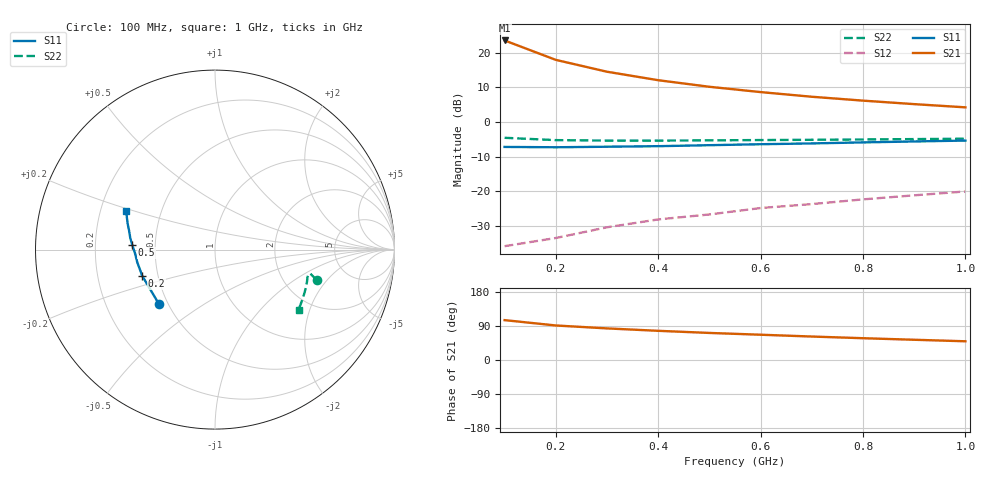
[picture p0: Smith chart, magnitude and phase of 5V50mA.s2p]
#  HZ  S  MA  R  50.0000
! Device:15GN03CA
! "! Bias:VCE=5V, IC=50mA  "
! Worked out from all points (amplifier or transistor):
!   10 points, 100 MHz to 1 GHz, reference 50 ohm
!   highest |S21| = 23.6 dB at 100 MHz (marker M1)
!   |S21| within 3 dB of that: start of sweep to 153.4 MHz
!   unconditionally stable (mu >= 1): start of sweep to end of sweep
!   at 200 MHz: K = 1.60, MAG = 21.2 dB, |S12| = -33.6 dB
!   at 600 MHz: K = 1.57, MAG = 12.3 dB, |S12| = -24.9 dB
!   at 1 GHz: K = 1.26, MAG = 9.1 dB, |S12| = -20.1 dB
!   S11 on the Smith chart (normalised r, x): 100 MHz: 0.45, -0.34; 200 MHz: 0.41, -0.15; 500 MHz: 0.37, +0.02; 1 GHz: 0.31, +0.19
1e8  0.436 -135.5  15.11 105.2  0.016 53.2  0.591 -16.6
2e8  0.431 -160.2  7.915 91.1  0.021 62.8  0.547 -14.1
3e8  0.439 -170.9  5.332 83.4  0.03 71.6  0.538 -15.1
4e8  0.447 -177.9  4.022 77.0  0.039 75.4  0.538 -16.9
5e8  0.462 176.8  3.231 71.4  0.046 77.8  0.543 -19.3
6e8  0.477 172.0  2.708 66.7  0.057 81.2  0.548 -22.4
7e8  0.49 167.6  2.318 61.9  0.065 82.5  0.553 -25.4
8e8  0.507 163.6  2.037 57.5  0.076 84.1  0.559 -28.7
9e8  0.523 159.9  1.813 53.4  0.087 86.2  0.566 -32.5
1e9  0.539 156.3  1.629 49.4  0.099 87.1  0.573 -35.7
